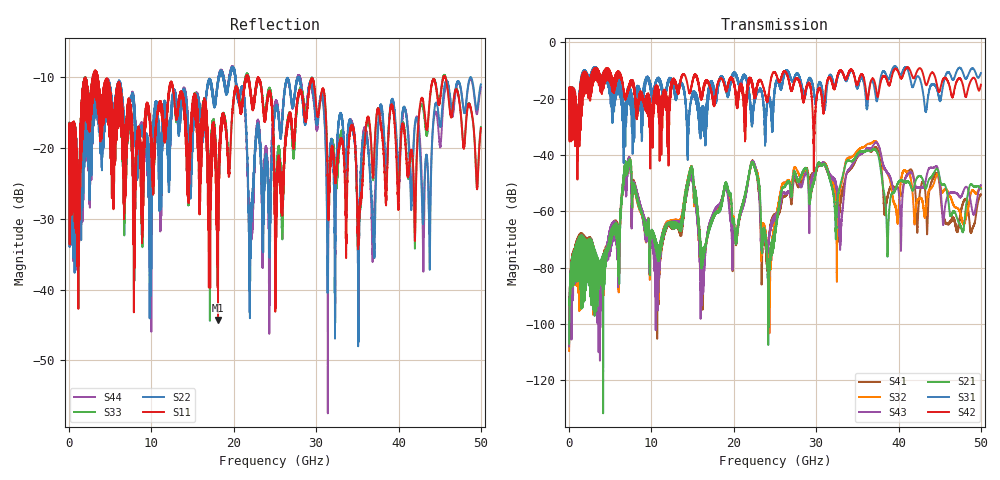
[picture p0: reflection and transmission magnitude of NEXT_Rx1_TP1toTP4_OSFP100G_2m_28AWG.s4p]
! Touchstone data
! Created: 27-Feb-2019 by IdEM 12 (12.1.0)
! COMMENTS
!  Created Wed Feb 27 12:03:36 2019
!  64 Port Network Data from SP1.SP block
!  freq  magS1_1  angS1_1  magS1_2  angS1_2  magS1_3  angS1_3  magS1_4  angS1_4
!  magS1_5  angS1_5  magS1_6  angS1_6  magS1_7  angS1_7  magS1_8  angS1_8
!  magS1_9  angS1_9  magS1_10  angS1_10  magS1_11  angS1_11  magS1_12  angS1_12
!  magS1_13  angS1_13  magS1_14  angS1_14  magS1_15  angS1_15  magS1_16  angS1_16
!  magS1_17  angS1_17  magS1_18  angS1_18  magS1_19  angS1_19  magS1_20  angS1_20
!  magS1_21  angS1_21  magS1_22  angS1_22  magS1_23  angS1_23  magS1_24  angS1_24
!  magS1_25  angS1_25  magS1_26  angS1_26  magS1_27  angS1_27  magS1_28  angS1_28
!  magS1_29  angS1_29  magS1_30  angS1_30  magS1_31  angS1_31  magS1_32  angS1_32
!  magS1_33  angS1_33  magS1_34  angS1_34  magS1_35  angS1_35  magS1_36  angS1_36
!  magS1_37  angS1_37  magS1_38  angS1_38  magS1_39  angS1_39  magS1_40  angS1_40
!  magS1_41  angS1_41  magS1_42  angS1_42  magS1_43  angS1_43  magS1_44  angS1_44
!  magS1_45  angS1_45  magS1_46  angS1_46  magS1_47  angS1_47  magS1_48  angS1_48
!  magS1_49  angS1_49  magS1_50  angS1_50  magS1_51  angS1_51  magS1_52  angS1_52
!  magS1_53  angS1_53  magS1_54  angS1_54  magS1_55  angS1_55  magS1_56  angS1_56
!  magS1_57  angS1_57  magS1_58  angS1_58  magS1_59  angS1_59  magS1_60  angS1_60
!  magS1_61  angS1_61  magS1_62  angS1_62  magS1_63  angS1_63  magS1_64  angS1_64
!  magS2_1  angS2_1  magS2_2  angS2_2  magS2_3  angS2_3  magS2_4  angS2_4
!  magS2_5  angS2_5  magS2_6  angS2_6  magS2_7  angS2_7  magS2_8  angS2_8
!  magS2_9  angS2_9  magS2_10  angS2_10  magS2_11  angS2_11  magS2_12  angS2_12
!  magS2_13  angS2_13  magS2_14  angS2_14  magS2_15  angS2_15  magS2_16  angS2_16
!  magS2_17  angS2_17  magS2_18  angS2_18  magS2_19  angS2_19  magS2_20  angS2_20
!  magS2_21  angS2_21  magS2_22  angS2_22  magS2_23  angS2_23  magS2_24  angS2_24
!  magS2_25  angS2_25  magS2_26  angS2_26  magS2_27  angS2_27  magS2_28  angS2_28
!  magS2_29  angS2_29  magS2_30  angS2_30  magS2_31  angS2_31  magS2_32  angS2_32
!  magS2_33  angS2_33  magS2_34  angS2_34  magS2_35  angS2_35  magS2_36  angS2_36
!  magS2_37  angS2_37  magS2_38  angS2_38  magS2_39  angS2_39  magS2_40  angS2_40
!  magS2_41  angS2_41  magS2_42  angS2_42  magS2_43  angS2_43  magS2_44  angS2_44
!  magS2_45  angS2_45  magS2_46  angS2_46  magS2_47  angS2_47  magS2_48  angS2_48
!  magS2_49  angS2_49  magS2_50  angS2_50  magS2_51  angS2_51  magS2_52  angS2_52
!  magS2_53  angS2_53  magS2_54  angS2_54  magS2_55  angS2_55  magS2_56  angS2_56
!  magS2_57  angS2_57  magS2_58  angS2_58  magS2_59  angS2_59  magS2_60  angS2_60
!  magS2_61  angS2_61  magS2_62  angS2_62  magS2_63  angS2_63  magS2_64  angS2_64
!  magS3_1  angS3_1  magS3_2  angS3_2  magS3_3  angS3_3  magS3_4  angS3_4
!  magS3_5  angS3_5  magS3_6  angS3_6  magS3_7  angS3_7  magS3_8  angS3_8
!  magS3_9  angS3_9  magS3_10  angS3_10  magS3_11  angS3_11  magS3_12  angS3_12
!  magS3_13  angS3_13  magS3_14  angS3_14  magS3_15  angS3_15  magS3_16  angS3_16
!  magS3_17  angS3_17  magS3_18  angS3_18  magS3_19  angS3_19  magS3_20  angS3_20
!  magS3_21  angS3_21  magS3_22  angS3_22  magS3_23  angS3_23  magS3_24  angS3_24
!  magS3_25  angS3_25  magS3_26  angS3_26  magS3_27  angS3_27  magS3_28  angS3_28
!  magS3_29  angS3_29  magS3_30  angS3_30  magS3_31  angS3_31  magS3_32  angS3_32
!  magS3_33  angS3_33  magS3_34  angS3_34  magS3_35  angS3_35  magS3_36  angS3_36
!  magS3_37  angS3_37  magS3_38  angS3_38  magS3_39  angS3_39  magS3_40  angS3_40
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# Hz S MA R 50
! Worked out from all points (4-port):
!   5000 points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, 10 MHz to 50 GHz, reference 50 ohm
!   strongest paths, dB at 10 MHz, 12.51 GHz, 25.01 GHz, 37.51 GHz, 50 GHz:
!     S42: -18.0, -13.6, -10.8, -19.3, -15.1
!     S31: -18.0, -14.0, -15.8, -18.9, -11.0
!     S21: -107.0, -65.6, -69.0, -40.0, -52.0
!     S43: -108.0, -65.0, -62.7, -36.2, -50.7
!     S32: -109.5, -64.5, -65.5, -36.3, -51.6
!     S41: -106.2, -66.2, -62.1, -38.3, -54.0
!   lowest |S11| = -44.3 dB at 18.09 GHz (marker M1), VSWR 1.01, Z = 49.5 + j0.362 ohm
!   |S11| at or under -10 dB: 3.49 GHz to 21.47 GHz (17.98 GHz wide, 144 % of centre); 21.77 GHz to 45.47 GHz (23.7 GHz wide, 70.5 % of centre); 45.66 GHz to end of sweep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
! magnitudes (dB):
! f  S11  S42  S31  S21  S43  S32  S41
! 10 MHz  -17.7  -18.0  -18.0  -107.0  -108.0  -109.5  -106.2
! 7.29 GHz  -13.7  -15.0  -16.2  -43.1  -41.5  -42.2  -42.3
! 10.66 GHz  -15.7  -19.2  -13.6  -75.7  -80.1  -85.7  -87.3
! 14.76 GHz  -18.0  -17.0  -21.8  -45.9  -48.3  -46.5  -47.5
! 16.18 GHz  -18.4  -19.6  -24.9  -75.6  -84.6  -76.7  -78.1
! 18.09 GHz  -44.3  -14.2  -16.7  -60.6  -58.2  -59.8  -58.7
! 50 GHz  -17.2  -15.1  -11.0  -52.0  -50.7  -51.6  -54.0
